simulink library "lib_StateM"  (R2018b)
settings: Solver=VariableStepAuto  StartTime=0.0  StopTime=10.0  RelTol=1e-3

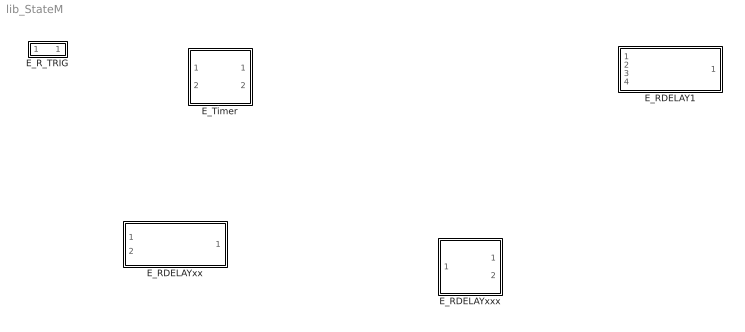
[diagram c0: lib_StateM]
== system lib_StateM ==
  E_RDELAY1 : Subsystem
  E_RDELAYxx : Subsystem  TreatAsAtomicUnit=on
  E_RDELAYxxx : Stateflow chart  TreatAsAtomicUnit=on
  E_R_TRIG : Stateflow chart  TreatAsAtomicUnit=on
  E_Timer : Stateflow chart  TreatAsAtomicUnit=on

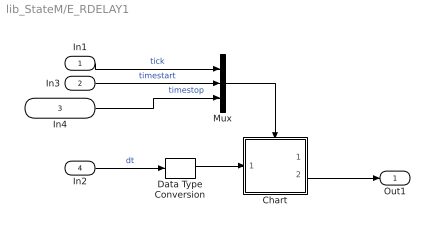
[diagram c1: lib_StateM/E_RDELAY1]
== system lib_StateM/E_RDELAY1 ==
  In1 : Inport
  In3 : Inport  Port=2
  In4 : Inport  Port=3
  In2 : Inport  Port=4  OutDataTypeStr=single
  Chart : Stateflow chart  TreatAsAtomicUnit=on
  Data Type Conversion : DataTypeConversion  OutDataTypeStr=uint32
  Mux : Mux  Inputs=3
  Out1 : Outport
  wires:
  In3/1 -> Mux/2  "timestart"
  In4/1 -> Mux/3  "timestop"
  Mux/1 -> Chart/Trigger
  Chart/2(tm()) -> Out1/1
  Data Type Conversion/1 -> Chart/1(dt)
  In2/1 -> Data Type Conversion/1  "dt"
  In1/1 -> Mux/1  "tick"

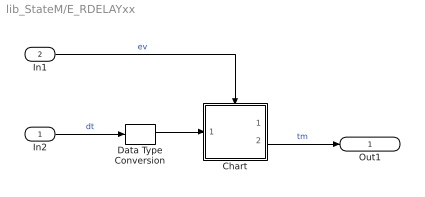
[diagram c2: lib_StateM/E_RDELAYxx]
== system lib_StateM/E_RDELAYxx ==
  In2 : Inport  OutDataTypeStr=single
  In1 : Inport  Port=2
  Chart : Stateflow chart  TreatAsAtomicUnit=on
  Data Type Conversion : DataTypeConversion  OutDataTypeStr=uint32
  Out1 : Outport
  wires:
  Chart/2(tm()) -> Out1/1  "tm"
  In2/1 -> Data Type Conversion/1  "dt"
  Data Type Conversion/1 -> Chart/1(dt)
  In1/1 -> Chart/Trigger  "ev"

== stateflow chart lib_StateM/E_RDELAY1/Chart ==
  state idle
  state counting
    entry: ct+=1;
  (default) -> idle
  idle -> counting : timestart/{ ct=0; }
  counting -> counting : tick[ct < dt]
  counting -> idle : timestop
  counting -> idle : tick[ct >= dt]/tm
  data: dt input uint32; ct output uint32
  events: input RISING_EDGE_EVENT; input RISING_EDGE_EVENT; output FUNCTION_CALL_EVENT; input RISING_EDGE_EVENT

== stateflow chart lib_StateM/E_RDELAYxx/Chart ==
  state idle
  state counting
    entry: ct+=1;
  (default) -> idle
  idle -> counting : timestart/{ ct=0; }
  counting -> counting : tick[ct < dt]
  counting -> idle : timestop
  counting -> idle : tick[ct >= dt]/tm
  data: dt input uint32; ct output uint32
  events: input RISING_EDGE_EVENT; input RISING_EDGE_EVENT; output FUNCTION_CALL_EVENT; input FUNCTION_CALL_EVENT

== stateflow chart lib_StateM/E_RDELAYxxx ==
  state idle
  state counting
    entry: ct+=1;
  (default) -> idle
  idle -> counting : timestart/{ ct=0; }
  counting -> counting : tick[ct < dt]
  counting -> idle : timestop
  counting -> idle : tick[ct >= dt]/tm
  data: dt input uint32; ct output uint32
  events: input FUNCTION_CALL_EVENT; input FUNCTION_CALL_EVENT; output FUNCTION_CALL_EVENT; input FUNCTION_CALL_EVENT

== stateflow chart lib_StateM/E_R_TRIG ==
  state b0
  state b1
    entry: ev
  (default) -> b0
  b0 -> b1 : [b]
  b1 -> b0 : [~b]
  data: b input boolean
  events: output FUNCTION_CALL_EVENT

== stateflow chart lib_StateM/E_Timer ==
  state idle
    entry: ct=0;
  state counting
    entry: ct +=Tstep;
  (default) -> idle
  idle -> counting : [dt>0]
  counting -> idle : [dt==0]
  counting -> counting : [ct < dt]
  counting -> idle : [dt >0 && ct >= dt] / tm
  data: dt input single; ct output single; Tstep input
  events: output FUNCTION_CALL_EVENT
